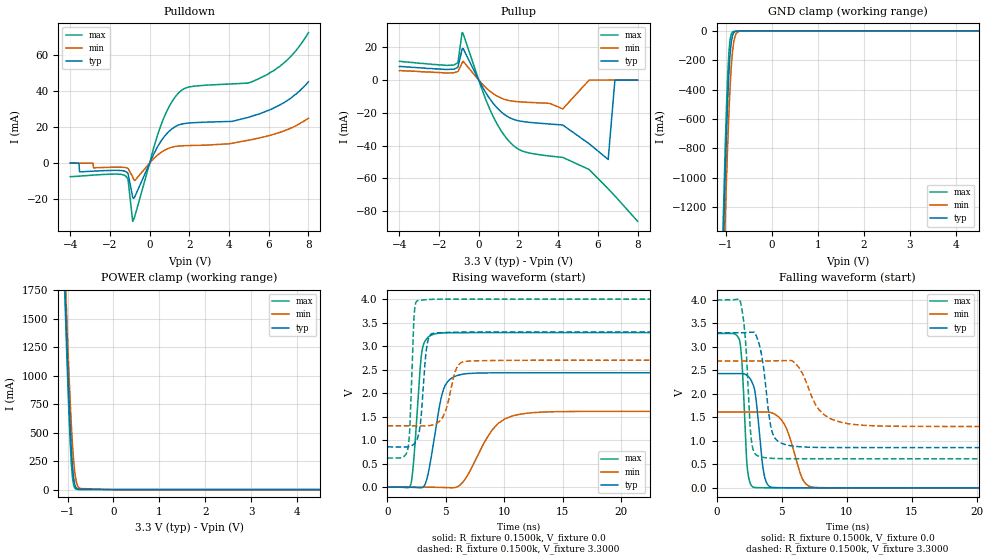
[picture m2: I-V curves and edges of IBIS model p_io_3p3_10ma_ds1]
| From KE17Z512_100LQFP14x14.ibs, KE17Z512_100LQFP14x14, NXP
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[Model] p_io_3p3_10ma_ds1
|   Model p_io_3p3_10ma_ds1
| This model was characterised for following simulation conditions:
| External (pad) voltage:
|   - Typ: 3.3V,   - Min: 2.7V,   - Max: 4.0V
| Library cells for typ/min/max conditions are connected as defined below:
|  pad - External Pad
|  ipp_do_lv - Core Input
|  ipp_obe_lv - Output Buffer Enable
|  abt_close_nor_rst_mv - vdde
|  dvdd - dvdd
|  dvss - dvss
|  esd_boost - vdde
|  ipp_dse_lv - dvdd
|  ipp_ina_280_mv - NC
|  ipp_ina_40_a_mv - NC
|  ipp_ina_40_b_mv - NC
|  ipp_ina_40_c_mv - NC
|  ipp_ina_40_d_mv - NC
|  ipp_ina_40_e_mv - NC
|  ipp_ina_40_f_mv - NC
|  ipp_ina_40_g_mv - NC
|  ipp_ina_40_h_mv - NC
|  ipp_ind_lv - NC
|  ipp_sre_lv - dvss
|  vdde - vdde
|  vsse - vsse
| All other pins connected to ground
Model_type I/O
Polarity   Non-Inverting
Enable   Active-High
Vinl =   0.9900V
Vinh =   2.3100V
Vmeas =  1.6500V
Cref =   50.0000F
C_comp   1.9352pF   1.8468pF   2.0590pF
[Model Spec]
| variable   typ   min   max
Vinh   2.3100V   1.8900V   2.8000V
Vinl   0.9900V   0.8100V   1.2000V
S_overshoot_high   3.6000V   3.0000V   4.3000V
S_overshoot_low   -0.3000V   -0.3000V   -0.3000V
Vmeas   1.6500V   1.3500V   2.0000V
[Temperature Range]   25.0000   0.1250k   -40.0000
[Voltage Range]   3.3000V   2.7000V   4.0000V
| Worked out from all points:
|   slope of the pulldown table from 0 to 0.495 V, typ, clamps not added: 45.6 ohm
|   slope of the pullup table from 0 to 0.495 V, typ, clamps not added: 47.9 ohm
|   rising waveform, R_fixture 0.1500k, V_fixture 0.0: 20-80 % time 1ns typ, 2.22ns min, 557ps max; typ from 0 V to 2.43 V
|   rising waveform, R_fixture 0.1500k, V_fixture 3.3000: 20-80 % time 464ps typ, 836ps min, 293ps max; typ from 0.857 V to 3.3 V
|   falling waveform, R_fixture 0.1500k, V_fixture 0.0: 20-80 % time 535ps typ, 1.09ns min, 340ps max; typ from 2.43 V to 0 V
|   falling waveform, R_fixture 0.1500k, V_fixture 3.3000: 20-80 % time 671ps typ, 1.53ns min, 418ps max; typ from 3.3 V to 0.857 V
[Pulldown]
|Voltage   I(typ)   I(min)   I(max)
-4V       0A         10uA       -7.52mA
-3.558V   -30uA      10uA       -7.21mA
-3.532V   -4.85mA    20uA       -7.19mA
-1.218V   -4.599mA   -2.451mA   -7.053mA
-1.088V   -5.751mA   -2.907mA   -9.093mA
-854mV    -18.79mA   -7.618mA   -32.27mA
-750mV    -18.71mA   -9.652mA   -29.65mA
550mV     11.84mA    5.811mA    20.5mA
1.434V    21.07mA    9.466mA    38.7mA
5.464V    27.1mA     13.8mA     46.72mA
6.894V    34.5mA     18.4mA     56.9mA
8V        45.2mA     24.9mA     72.5mA
[Pullup]
|Voltage   I(typ)   I(min)   I(max)
-4V       8.3mA      5.8mA      11.5mA
-1.256V   6.69mA     4.49mA     9.21mA
-1.048V   8.03mA     5.34mA     11mA
-814mV    19.34mA    11.14mA    28.9mA
538mV     -11.14mA   -6.546mA   -17.3mA
1.552V    -22.94mA   -12.55mA   -37.69mA
2.332V    -25.48mA   -13.47mA   -43.87mA
4.23V     -27.44mA   -17.57mA   -47.21mA
5.556V    -38.82mA   -10uA      -54.56mA
6.518V    -48.48mA   10uA       -66.38mA
6.856V    -30uA      20uA       -70.73mA
8V        30uA       20uA       -86.22mA
[GND_clamp]
|Voltage   I(typ)   I(min)   I(max)
-4V       -44.22A    -44.15A    -44.31A
-1.062V   -1.538A    -1.84A     -1.36A
-1.036V   -1.238A    -1.547A    -1.053A
-1.01V    -956.2mA   -1.268A    -766.3mA
-958mV    -472.3mA   -768mA     -297.7mA
-932mV    -288.7mA   -557.4mA   -144.7mA
-906mV    -155.5mA   -380.4mA   -57.41mA
-880mV    -73.51mA   -241.5mA   -20.32mA
-828mV    -13.22mA   -77.7mA    -4.19mA
-776mV    -3.062mA   -20.44mA   -2.572mA
-698mV    -1.117mA   -2.814mA   -1.68mA
8V        0A         0A         0A
[POWER_clamp]
|Voltage   I(typ)   I(min)   I(max)
-4V       44.89A     44.69A     45.07A
-1.074V   1.999A     2.184A     1.905A
-1.048V   1.679A     1.877A     1.575A
-1.022V   1.371A     1.58A      1.256A
-970mV    807.7mA    1.033A     674.4mA
-918mV    359.9mA    574.8mA    234.3mA
-892mV    203mA      392.8mA    103.5mA
-866mV    99.48mA    249.2mA    36.93mA
-814mV    17.16mA    79.21mA    3.9mA
-736mV    1.301mA    9.822mA    753.1uA
0V        71.73pA    1.381nA    67.44pA
8V        0A         0A         0A
[Ramp]
| variable   typ   min   max
dV/dt_r  1.4597/1.0002n   0.9678/2.2159n   1.9721/0.5574n
dV/dt_f  1.4659/0.6708n   0.8362/1.5330n   2.0283/0.4180n
R_load = 0.1500k
[Rising Waveform]
R_fixture= 0.1500k
V_fixture= 0.0
V_fixture_min= 0.0
V_fixture_max= 0.0
|time   V(typ)   V(min)   V(max)
0s        55.35pV    15.57nV    185.3pV
2.002ns   -2.948mV   65.27uV    58.54mV
2.256ns   -4.984mV   79.5uV     588.3mV
2.942ns   -13.11mV   -15.13uV   2.877V
3.908ns   884.5mV    -2.158mV   3.251V
4.803ns   2.085V     -7.521mV   3.282V
6.48ns    2.404V     115.1mV    3.287V
8.94ns    2.432V     1.209V     3.287V
11.22ns   2.433V     1.546V     3.287V
40ns      2.433V     1.613V     3.287V
[Rising Waveform]
R_fixture= 0.1500k
V_fixture= 3.3000
V_fixture_min= 2.7000
V_fixture_max= 4.0000
|time   V(typ)   V(min)   V(max)
0s        856.8mV    1.306V     619.5mV
1.794ns   859.6mV    1.305V     877.7mV
1.919ns   866.8mV    1.305V     1.287V
2.255ns   912.3mV    1.304V     3.54V
2.573ns   1.038V     1.303V     3.966V
2.833ns   1.376V     1.302V     3.977V
3.334ns   2.929V     1.303V     3.989V
3.895ns   3.272V     1.324V     3.996V
6.721ns   3.299V     2.677V     4V
40ns      3.3V       2.7V       4V
[Falling Waveform]
R_fixture= 0.1500k
V_fixture= 0.0
V_fixture_min= 0.0
V_fixture_max= 0.0
|time   V(typ)   V(min)   V(max)
0s        2.433V     1.613V     3.287V
1.79ns    2.435V     1.613V     3.116V
1.986ns   2.433V     1.613V     2.5V
2.371ns   2.387V     1.613V     391.2mV
2.894ns   2.122V     1.613V     8.181mV
3.619ns   328mV      1.616V     1.628mV
4.253ns   11.48mV    1.595V     592.8uV
5.209ns   2.075mV    1.354V     145.2uV
7.312ns   180.5uV    18.48mV    16.22uV
40ns      1.359uV    2.761uV    626.3nV
[Falling Waveform]
R_fixture= 0.1500k
V_fixture= 3.3000
V_fixture_min= 2.7000
V_fixture_max= 4.0000
|time   V(typ)   V(min)   V(max)
0s        3.3V       2.7V       4V
1.796ns   3.3V       2.7V       4.003V
2.214ns   3.305V     2.7V       3.168V
2.649ns   3.313V     2.7V       1.068V
3.301ns   3.028V     2.7V       667.3mV
4.282ns   1.178V     2.703V     627.8mV
5.61ns    900.1mV    2.711V     620.4mV
7.851ns   860.6mV    1.671V     619.6mV
10.07ns   857.3mV    1.367V     619.5mV
40ns      856.8mV    1.306V     619.5mV
